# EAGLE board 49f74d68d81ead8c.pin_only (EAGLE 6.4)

Size 27.64 x 57.71 mm. Coordinates in mm from the lower left corner, seen from the top.
Outline: 19.81,0 25.09,0 arc90 27.64,2.54 27.64,55.17 arc90 25.09,57.71 2.54,57.71 arc90 0,55.17 0,2.54 arc90 2.54,0 6.1,0 arc90 8.13,2.03 17.78,2.03 arc90 19.81,0
Copper layers (1*16): Top 0.035mm / dielectric 1.5mm / Bottom 0.035mm
Design rules "adafruit *": minimum track width 8mil, minimum drill 15.5mil, track to track 8mil, track to pad 8mil, pad to pad 8mil, via to via 8mil, smd to smd 8mil, copper to edge 10mil, drill to drill 8mil, minimum pad ring 10mil, minimum via ring 8mil, stop-mask expansion 4mil, vias tented up to drill 20mil, thermal gap 10mil

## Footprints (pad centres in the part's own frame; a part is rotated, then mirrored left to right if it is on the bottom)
PANASONIC_C = smd 2.6 x 1.4: + 2.05,0; - -2.05,0
_0805MP = smd 1.2 x 1.3: 1 -1.016,0; 2 1.016,0
MICROSD = smd 0.7 x 1.5: 1 9,-10.64; 2 7.9,-10.24; 3 6.8,-10.64; 4 5.7,-11.04; 5 4.6,-10.64; 6 3.5,-11.04; 7 2.4,-10.64; 8 1.3,-10.64 | smd 1.8 x 1.4: CD1 2,-0.44; CD2 8,-0.44 | smd 1.4 x 1.9: MT1 0.4,-13.54; MT2 13.6,-14.44
SOD-323 = smd 1.35 x 0.8: A 1.27,0; C -1.27,0
FIDUCIAL_1MM = smd 1 x 1: 1 0,0
1X16_ROUND = drill 1 pad 1.676: 1 -19.05,0; 2 -16.51,0; 3 -13.97,0; 4 -11.43,0; 5 -8.89,0; 6 -6.35,0; 7 -3.81,0; 8 -1.27,0; 9 1.27,0; 10 3.81,0; 11 6.35,0; 12 8.89,0; 13 11.43,0; 14 13.97,0; 15 16.51,0; 16 19.05,0
RESPACK_4X0603 = smd 0.45 x 0.9: 1 -1.3,-0.85; 2 -0.4,-0.85; 3 0.4,-0.85; 4 1.3,-0.85; 5 1.3,0.85; 6 0.4,0.85; 7 -0.4,0.85; 8 -1.3,0.85
0805-NO = smd 1.3 x 1.5: 1 -0.95,0; 2 0.95,0
LQFP48 = smd 1.1 x 0.285: 1 -4.2,2.75; 2 -4.2,2.25; 3 -4.2,1.75; 4 -4.2,1.25; 5 -4.2,0.75; 6 -4.2,0.25; 7 -4.2,-0.25; 8 -4.2,-0.75; 9 -4.2,-1.25; 10 -4.2,-1.75; 11 -4.2,-2.25; 12 -4.2,-2.75; 25 4.2,-2.75; 26 4.2,-2.25; 27 4.2,-1.75; 28 4.2,-1.25; 29 4.2,-0.75; 30 4.2,-0.25; 31 4.2,0.25; 32 4.2,0.75; 33 4.2,1.25; 34 4.2,1.75; 35 4.2,2.25; 36 4.2,2.75 | smd 0.285 x 1.1: 13 -2.75,-4.2; 14 -2.25,-4.2; 15 -1.75,-4.2; 16 -1.25,-4.2; 17 -0.75,-4.2; 18 -0.25,-4.2; 19 0.25,-4.2; 20 0.75,-4.2; 21 1.25,-4.2; 22 1.75,-4.2; 23 2.25,-4.2; 24 2.75,-4.2; 37 2.75,4.2; 38 2.25,4.2; 39 1.75,4.2; 40 1.25,4.2; 41 0.75,4.2; 42 0.25,4.2; 43 -0.25,4.2; 44 -0.75,4.2; 45 -1.25,4.2; 46 -1.75,4.2; 47 -2.25,4.2 | smd 0.28 x 1.1: 48 -2.75,4.2
SOT23-6 = smd 0.55 x 1.2: 1 -0.95,-1.3; 2 0,-1.3; 3 0.95,-1.3; 4 0.95,1.3; 5 0,1.3; 6 -0.95,1.3
SOIC16 = smd 0.6 x 2.2: 1 -4.445,-2.6; 2 -3.175,-2.6; 3 -1.905,-2.6; 4 -0.635,-2.6; 5 0.635,-2.6; 6 1.905,-2.6; 7 3.175,-2.6; 8 4.445,-2.6; 9 4.445,2.6; 10 3.175,2.6; 11 1.905,2.6; 12 0.635,2.6; 13 -0.635,2.6; 14 -1.905,2.6; 15 -3.175,2.6; 16 -4.445,2.6
MOUNTINGHOLE_3.0_PLATEDTHIN = drill 3 pad 3.6: P$1 0,0
CRYSTAL_3.2X2.5 = smd 1.4 x 1.2: 1 -1.1,-0.8; 2 1.1,0.8; GND1 -1.1,0.8; GND2 1.1,-0.8

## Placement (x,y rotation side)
C1  220uF  [PANASONIC_C]  18.54,51.56 270 top
C2  220uF  [PANASONIC_C]  12.7,51.56 270 top
C4  10pF  [_0805MP]  15.62,31.52 270 top
C5  10pF  [_0805MP]  12.62,29.08 0 top
C6  10µF  [_0805MP]  18.41,27.56 270 top
C7  10µF  [_0805MP]  20.07,27.56 270 top
C8  0.1µF  [_0805MP]  9.19,45.76 0 top
C19  10µF  [_0805MP]  3.3,8.64 0 top
C20  10µF  [_0805MP]  19.53,34.21 180 top
C21  10nF (0.01uF)  [_0805MP]  7.2,51.66 180 top
C22  10nF (0.01uF)  [_0805MP]  18.95,45.37 180 top
C26  0.1µF  [_0805MP]  5.38,39.43 270 top
CN1  2908-05WB-M6  [MICROSD]  6.36,16 0 top
D1  1N4148  [SOD-323]  5.97,20.83 270 top
FB1  FERITTE  [_0805MP]  6.66,48.77 270 top
FB2  FERITTE  [_0805MP]  22.32,38.55 180 top
FID1  FIDUCIAL""  [FIDUCIAL_1MM]  5.71,56.52 0 top
FID2  FIDUCIAL""  [FIDUCIAL_1MM]  22.04,1.22 0 top
JP2  [1X16_ROUND]  25.4,30.48 270 top
JP3  [1X16_ROUND]  2.54,30.48 270 top
R1  1M  [_0805MP]  13.49,34.19 0 top
R2  100K  [_0805MP]  5.31,43.49 0 top
R3  20  [_0805MP]  8.73,48.83 90 top
R4  20  [_0805MP]  18.87,47.14 0 top
R6  100  [_0805MP]  15.91,47.77 270 top
R7  100  [_0805MP]  12.86,47.01 180 top
R8  100K  [RESPACK_4X0603]  6.5,26.49 270 top
R9  100K  [RESPACK_4X0603]  21.01,19.05 270 top
R10  10K  [0805-NO]  5.46,17.78 180 top
R16  100K  [RESPACK_4X0603]  6.43,34.11 270 top
U1  VS1053B  [LQFP48]  13.97,40.77 0 top
U2  AP7312-1833W6-7  [SOT23-6]  19.57,31.12 90 top
U3  74HC4050D  [SOIC16]  13.39,21.84 180 top
U$31  [ADAFRUIT_3.5MM]  6.6,28.7 0 top
U$50  MOUNTINGHOLE3.0THIN  [MOUNTINGHOLE_3.0_PLATEDTHIN]  2.92,3.81 0 top
U$51  MOUNTINGHOLE3.0THIN  [MOUNTINGHOLE_3.0_PLATEDTHIN]  24.26,3.81 0 top
U$52  MOUNTINGHOLE3.0THIN  [MOUNTINGHOLE_3.0_PLATEDTHIN]  24.26,54.23 0 top
U$53  MOUNTINGHOLE3.0THIN  [MOUNTINGHOLE_3.0_PLATEDTHIN]  2.92,54.23 0 top
U$55  [ADAFRUIT_TEXT_20MM]  24.28,5.33 0 bottom
Y1  ABM8G-12.288MHZ-4Y-T3  [CRYSTAL_3.2X2.5]  12.79,31.64 0 top

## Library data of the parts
C1 C2 = rcl
C4-C8 C19-C22 C26 CN1 D1 FB1 FB2 JP2 JP3 R1-R4 R6-R10 R16 U1-U3 U$31 U$55 Y1 = microbuilder
FID1 FID2 U$50-U$53 = microbuilder; BOM: EXCLUDE

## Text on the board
tPlace: VS1053B AUDIO | v2 | ROUT | LINE2 | LOUT | MIC+ | AGND | MIC- | AGND | AGND | GND | 3V3 | DREQ | 0 | VCC | 1 | 3V3 | 2 | GND | 3 | MISO | 4 | MOSI | 5 | SCLK | 6 | 7 | RST | CS | TX | SDCS | RX | SD | XDCS | CD | 5V | SAFE
bPlace: OGG, MP3, AAC, WMA, FLAC, MIDI | VS1053B Audio Codec | 3.3V | 3.3 - 5V | OK for use w/powered speakers | LOUT/ROUT: 16Ω Stereo Headphone/Line Out | RX/TX SERIAL: 3-5V safe | SPI: 3-5V safe | GPIO: | VCC: | Supports:
